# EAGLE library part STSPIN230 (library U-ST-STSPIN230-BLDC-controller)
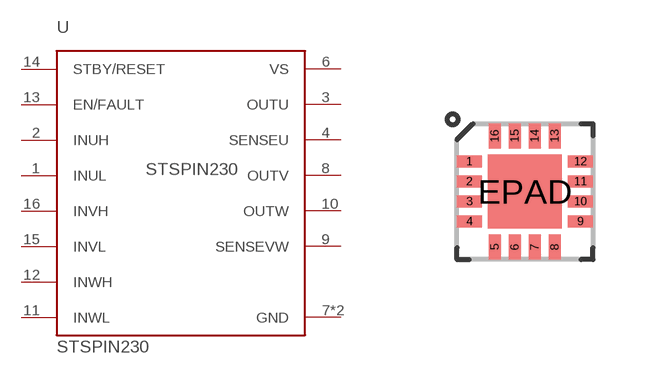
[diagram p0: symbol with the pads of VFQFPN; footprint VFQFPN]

Designator prefix U

## STSPIN230  [VFQFPN]
1  INUL  in
2  INUH  in
3  OUTU  out
4  SENSEU  out
6  VS  pwr
7  GND  pwr
8  OUTV  out
9  SENSEVW  out
10  OUTW  out
11  INWL  in
12  INWH  in
13  EN/FAULT
14  STBY/RESET  in
15  INVL  in
16  INVH  in
EPAD  GND  pwr

## Footprint VFQFPN (pad centres in mm)
smd 0.63 x 0.3: 1 -1.39,0.75; 2 -1.39,0.25; 3 -1.39,-0.25; 4 -1.39,-0.75; 9 1.39,-0.75; 10 1.39,-0.25; 11 1.39,0.25; 12 1.39,0.75
smd 0.3 x 0.63: 5 -0.75,-1.39; 6 -0.25,-1.39; 7 0.25,-1.39; 8 0.75,-1.39; 13 0.75,1.39; 14 0.25,1.39; 15 -0.25,1.39; 16 -0.75,1.39
smd 1.85 x 1.85: EPAD 0,0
